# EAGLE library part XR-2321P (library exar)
V.23/V.21 MODEM
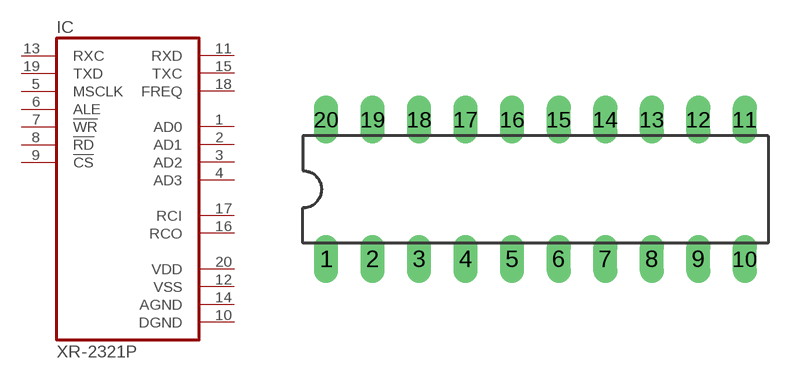
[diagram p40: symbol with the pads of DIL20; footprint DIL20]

Designator prefix IC

## XR-2321P (OC_FARNELL: unknown; OC_NEWARK: unknown)  [DIL20]
1  AD0
2  AD1
3  AD2
4  AD3
5  MSCLK  in
6  ALE  in
7  !WR  in
8  !RD  in
9  !CS  in
10  DGND  pwr
11  RXD  out
12  VSS  pwr
13  RXC  in
14  AGND  pwr
15  TXC  out
16  RCO
17  RCI
18  FREQ  out
19  TXD  in
20  VDD  pwr

## Footprint DIL20 (pad centres in mm)
Dual In Line Package
drill 0.813 long: 1 -11.43,-3.81; 2 -8.89,-3.81; 3 -6.35,-3.81; 4 -3.81,-3.81; 5 -1.27,-3.81; 6 1.27,-3.81; 7 3.81,-3.81; 8 6.35,-3.81; 9 8.89,-3.81; 10 11.43,-3.81; 11 11.43,3.81; 12 8.89,3.81; 13 6.35,3.81; 14 3.81,3.81; 15 1.27,3.81; 16 -1.27,3.81; 17 -3.81,3.81; 18 -6.35,3.81; 19 -8.89,3.81; 20 -11.43,3.81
